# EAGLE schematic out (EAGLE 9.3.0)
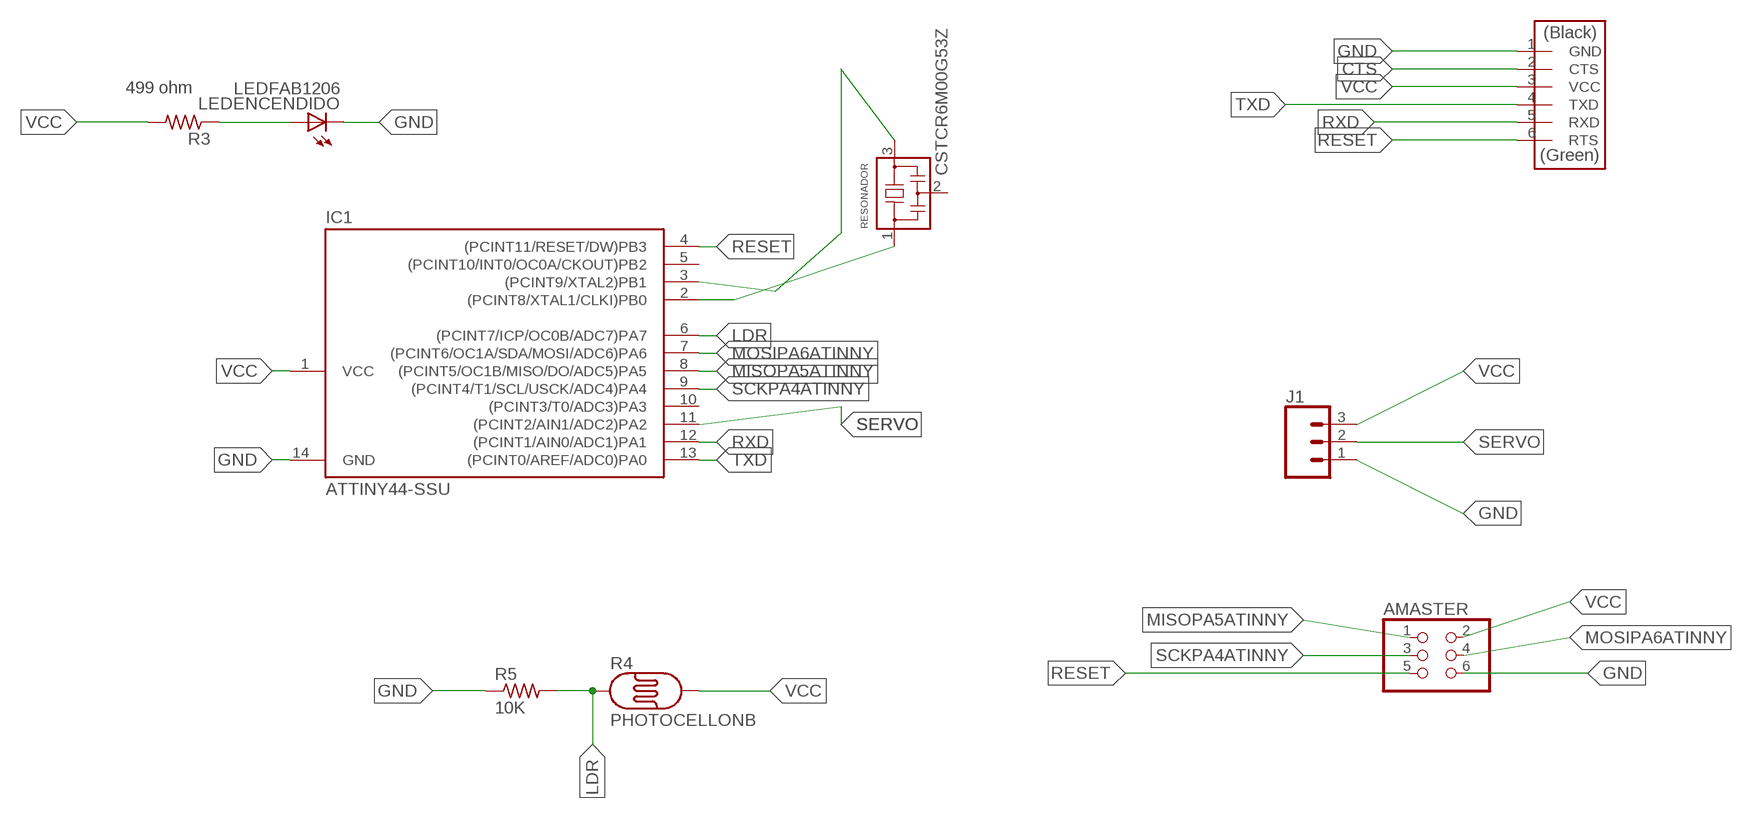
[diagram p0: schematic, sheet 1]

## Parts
AMASTER  PINHD-2X3-SMD  [2X03SMD]
IC1  ATTINY44-SSU  [SOIC14]
J1  CONN_031X03_SMD_RA_MALE_POST_SMALLER  [1X03_SMD_RA_MALE_POST_SMALLER]
J3  FTDI-SMD-HEADER  [1X06SMD]
LEDENCENDIDO  LEDFAB1206  [LED1206FAB]
R3  499 ohm  RES-US1206FAB  [R1206FAB]
R4  PHOTOCELLONB  [ON_BOARD]
R5  10K  RES-US1206FAB  [R1206FAB]
RESONADOR  CSTCR6M00G53Z  [CSTCR6M]

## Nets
CTS: J3.2(CTS)
GND: AMASTER.6 IC1.14(GND) J1.1 J3.1(GND) LEDENCENDIDO.2(C) R5.1
LDR: IC1.6((PCINT7/ICP/OC0B/ADC7)PA7) R4.1 R5.2
MISOPA5ATINNY: AMASTER.1 IC1.8((PCINT5/OC1B/MISO/DO/ADC5)PA5)
MOSIPA6ATINNY: AMASTER.4 IC1.7((PCINT6/OC1A/SDA/MOSI/ADC6)PA6)
N$1: LEDENCENDIDO.1(A) R3.1
RESET: AMASTER.5 IC1.4((PCINT11/RESET/DW)PB3) J3.6(RTS)
RXD: IC1.12((PCINT1/AIN0/ADC1)PA1) J3.5(RXD)
SCKPA4ATINNY: AMASTER.3 IC1.9((PCINT4/T1/SCL/USCK/ADC4)PA4)
SERVO: IC1.11((PCINT2/AIN1/ADC2)PA2) J1.2
TXD: IC1.13((PCINT0/AREF/ADC0)PA0) J3.4(TXD)
VCC: AMASTER.2 IC1.1(VCC) J1.3 J3.3(VCC) R3.2 R4.2
XTAL1: IC1.2((PCINT8/XTAL1/CLKI)PB0) RESONADOR.1
XTAL2: IC1.3((PCINT9/XTAL2)PB1) RESONADOR.3
Unconnected: IC1.5((PCINT10/INT0/OC0A/CKOUT)PB2) IC1.10((PCINT3/T0/ADC3)PA3) RESONADOR.2

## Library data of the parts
AMASTER = fab:PINHD-2X3-SMD: PIN HEADER
IC1 = fab:ATTINY44
J1 = SparkFun-Connectors:CONN_03: Multi connection point. Often used as Generic Header-pin footprint for 0.1 inch spaced/style header connections On any of the 0.1 inch spaced packages, you can populate with these: Break Away Headers - Straight (PRT-00116) Break Away Male Headers - Right Angle (PRT-00553) Female Headers (PRT-00115)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; PROD_ID: CONN-11912
J3 = fab:FTDI-SMD-HEADER
LEDENCENDIDO = fab:LED: LED
R3 R5 = fab:RES-US: Resistor (US Symbol)
R4 = ldr:PHOTOCELL: Photo Resitor
RESONADOR = murata-filter:CSTCR: Resonator Source: murata.co.jp; MPN: CSTCR6M00G53-R0; OC_FARNELL: 1170434; OC_NEWARK: 25M8759

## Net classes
0 default: clearance 0.205 mm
